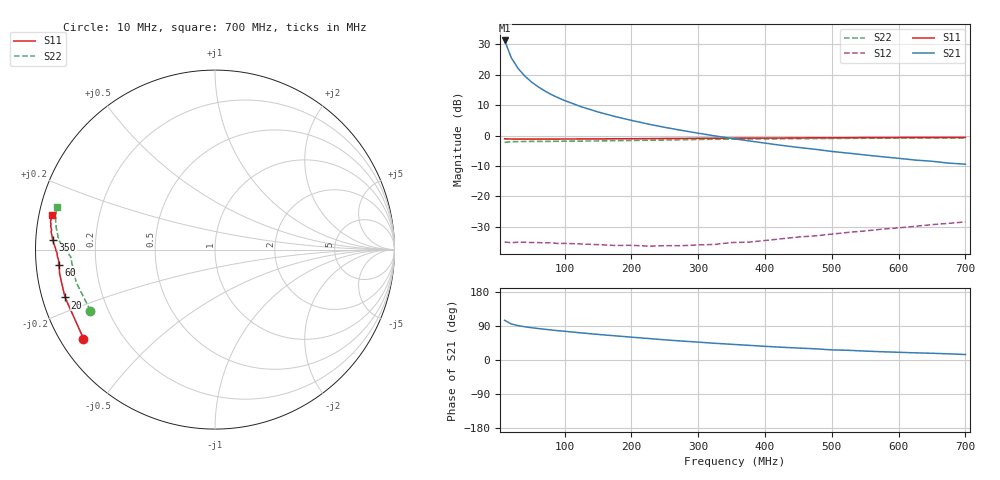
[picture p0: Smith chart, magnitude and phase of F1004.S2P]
! Date: Mon Aug 07 14:49:07 1995
# MHZ  S  MA  R  50.0000
!  POLYFET RF DEVICES
!  F1004
!  S PARAMETERS
!  VDS=28V, IDQ=800mA
!FREQ  S11MAG S11ANG S21MAG S21ANG S12MAG S12ANG S22MAG S22ANG
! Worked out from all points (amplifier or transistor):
!   34 points, 10 MHz to 700 MHz, reference 50 ohm
!   highest |S21| = 31.2 dB at 10 MHz (marker M1)
!   |S21| within 3 dB of that: start of sweep to 15.3 MHz
!   unconditionally stable (mu >= 1): 195.5 MHz to end of sweep
!   at 60 MHz: K = 0.30, MSG = 25.6 dB, |S12| = -35.1 dB
!   at 300 MHz: K = 1.33, MAG = 14.9 dB, |S12| = -35.9 dB
!   at 700 MHz: K = 1.04, MAG = 8.3 dB, |S12| = -28.3 dB
!   S11 on the Smith chart (normalised r, x): 10 MHz: 0.07, -0.31; 20 MHz: 0.07, -0.15; 60 MHz: 0.07, -0.05; 350 MHz: 0.05, +0.03; 700 MHz: 0.04, +0.10
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10  0.8847 -145.9  36.42 104.8  0.01791 19.7  0.7729 -153.9
20  0.8768 -162.3  18.98 95.0  0.01739 7.6  0.7946 -166.7
30  0.8745 -168.3  12.72 90.8  0.01776 7.6  0.796 -171.1
40  0.876 -171.4  9.537 87.7  0.01772 5.1  0.7987 -173.4
50  0.8738 -173.1  7.62 85.2  0.01753 5.2  0.8014 -174.8
60  0.8757 -174.5  6.336 83.1  0.01751 5.9  0.8018 -175.6
70  0.8738 -175.5  5.415 81.1  0.01725 6.4  0.7998 -176.3
80  0.8736 -176.3  4.715 79.3  0.01747 5.7  0.8031 -176.6
90  0.8759 -176.7  4.182 77.4  0.01687 6.7  0.8042 -177.2
100  0.8785 -177.3  3.753 75.8  0.01699 7.9  0.8079 -177.4
125  0.8794 -178.1  2.965 71.5  0.01657 9.4  0.8132 -178.0
150  0.8806 -179.0  2.439 67.5  0.01616 9.7  0.8141 -178.9
175  0.8868 -179.7  2.059 63.8  0.01569 11.9  0.8256 -179.5
200  0.8872 179.9  1.773 60.3  0.01576 16.8  0.8308 -179.9
225  0.8897 179.3  1.544 56.7  0.01527 18.3  0.8372 179.6
250  0.8938 178.7  1.363 53.2  0.01554 24.1  0.844 179.0
300  0.9007 177.6  1.092 47.2  0.01601 33.2  0.8618 177.5
350  0.9059 176.6  0.8974 41.4  0.01753 38.8  0.8701 176.1
375  0.9078 176.1  0.8203 38.8  0.01776 43.9  0.8772 175.4
475  0.9183 173.7  0.5949 29.5  0.02254 53.4  0.8937 172.1
600  0.9282 170.6  0.4227 20.4  0.03052 57.4  0.9082 167.9
700  0.9306 168.2  0.3387 14.5  0.03826 58.2  0.91 164.7
